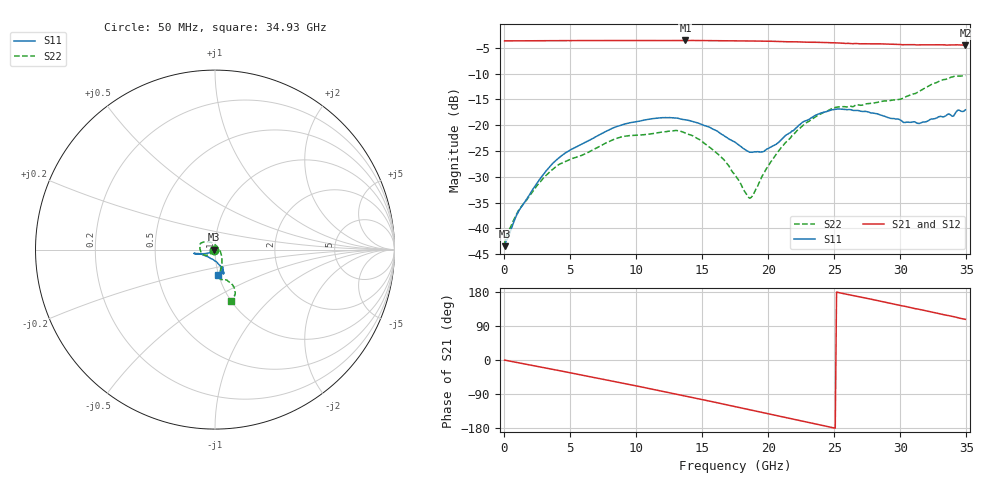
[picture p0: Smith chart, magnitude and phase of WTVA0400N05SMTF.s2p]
! 50 ohm 2-Port S-parameters measured by Modelithics Inc support@modelithics.com  Tampa, FL USA 813-866-6335 (February 2024)
! Smiths Interconnect,  4dB P/N: WTVA0400N05SMTF, Temperature: 50 C
! Board: 10 mil Rogers 4350B, Mounting Pad Dimensions: Length: 15 mils, Width: 25 mils, Gap: 40 mils.
# Hz S RI R 50
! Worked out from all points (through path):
!   352 points, 50 MHz to 34.93 GHz, reference 50 ohm
!   highest |S21| = -3.60 dB at 13.73 GHz (marker M1); lowest = -4.5 dB at 34.93 GHz (marker M2)
!   group delay of S21, straight-line fit = 20.3 ps
!   lowest |S11| = -43.4 dB at 50 MHz (marker M3), VSWR 1.01, Z = 49.3 - j0.00514 ohm
!   |S11| at or under -10 dB: start of sweep to end of sweep
!   |S22| runs from -43.1 to -10.4 dB; largest |S21 - S12| = 0.0075
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5e7  -0.00674 -5.21e-05  0.6543 -0.00327  0.6538 -0.00342  -0.00677 -0.00167
2e8  -0.00747 -0.00198  0.654 -0.0154  0.6535 -0.0154  -0.00821 -0.00256
1.0955e9  -0.0124 -0.00765  0.6493 -0.0829  0.6487 -0.0829  -0.0117 -0.00914
2.986e9  -0.0289 -0.0165  0.6169 -0.2225  0.6161 -0.2229  -0.0222 -0.0213
4.2795e9  -0.045 -0.0212  0.5773 -0.3151  0.5765 -0.3149  -0.032 -0.0277
5.8715e9  -0.0612 -0.0229  0.5079 -0.4198  0.5073 -0.4193  -0.0407 -0.0306
8.8565e9  -0.097 -0.024  0.3273 -0.572  0.3257 -0.572  -0.0729 -0.0241
1.1742e10  -0.1152 -0.0229  0.1078 -0.6502  0.1065 -0.6497  -0.0846 0.00943
1.3732e10  -0.1105 -0.021  -0.0576 -0.6581  -0.0583 -0.6574  -0.0748 0.0378
1.62195e10  -0.0828 -0.0233  -0.2606 -0.6034  -0.2611 -0.6026  -0.031 0.042
1.7513e10  -0.0596 -0.033  -0.3573 -0.5508  -0.3574 -0.55  -0.00732 0.0317
1.8508e10  -0.037 -0.0414  -0.4242 -0.4968  -0.4244 -0.496  0.0129 0.0153
1.8707e10  -0.0324 -0.0441  -0.4365 -0.4848  -0.4367 -0.4839  0.0165 0.0111
1.9702e10  -0.0115 -0.0547  -0.4945 -0.4223  -0.4944 -0.4215  0.0312 -0.0149
2.09955e10  0.0116 -0.0715  -0.5552 -0.3274  -0.5548 -0.327  0.0383 -0.0473
2.33835e10  0.0438 -0.112  -0.6192 -0.1417  -0.6186 -0.1417  0.0315 -0.1115
2.5274e10  0.0486 -0.135  -0.6249 0.0178  -0.6242 0.0175  0.0185 -0.1487
2.91545e10  0.0313 -0.113  -0.5281 0.3031  -0.5246 0.3075  0.0414 -0.1672
3.1443e10  0.0392 -0.0963  -0.413 0.433  -0.4105 0.4343  0.0935 -0.1916
3.3035e10  0.0445 -0.1133  -0.315 0.5101  -0.3104 0.512  0.1127 -0.2453
3.403e10  0.0315 -0.1185  -0.2481 0.5448  -0.2433 0.5462  0.107 -0.2758
3.49255e10  0.0179 -0.1395  -0.1774 0.567  -0.177 0.5661  0.0915 -0.2887
